(* SV publisher ASDU *)
{attribute 'analysis' := '-33'}
{attribute 'no_assign'}
{attribute 'no_explicit_call' := 'Direct call not allowed for type FB_SVTXASDU_IED_MUnn_LLN0_MSVCB01'}
FUNCTION_BLOCK FB_SVTXASDU_IED_MUnn_LLN0_MSVCB01 EXTENDS FB_GseSvAsduClass
VAR_INPUT
	Values: ST_SVDATA_IED_MUnn_LLN0_PhsMeas1; (* SV dataset values buffer in IEC 61850 network transfer format (big endian) *)
END_VAR
VAR
	bAdd: BOOL := THIS^.AddValuesToContainer(pValues:=ADR(Values), cbValues:=SIZEOF(Values)); (* Adds SV dataset values buffer to the ASDU *)
END_VAR

END_FUNCTION_BLOCK
